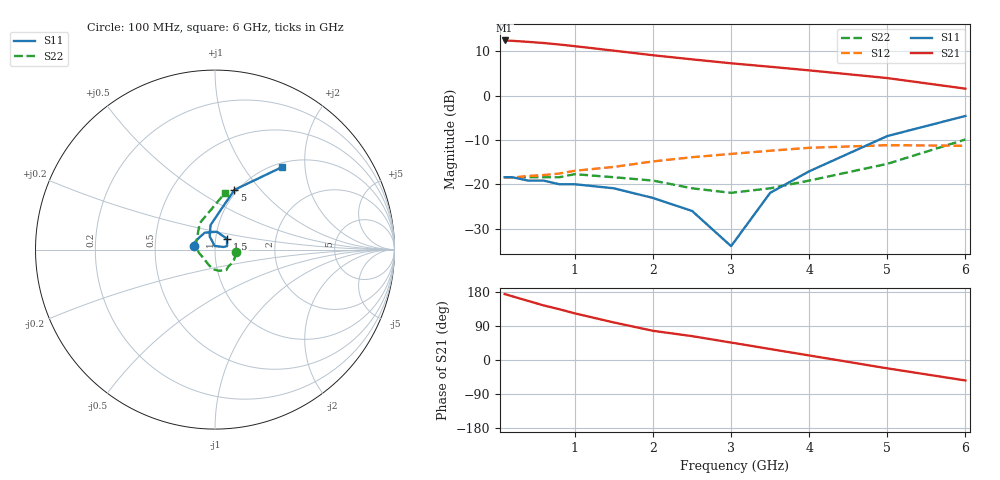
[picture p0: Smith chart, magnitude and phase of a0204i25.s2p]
!  MSA-0204 S AND NOISE PARAMETERS
!  Id=25mA  LAST UPDATED 07-22-92
# ghz s ma r 50
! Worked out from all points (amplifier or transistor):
!   14 points, 100 MHz to 6 GHz, reference 50 ohm
!   highest |S21| = 12.5 dB at 100 MHz (marker M1)
!   |S21| within 3 dB of that: start of sweep to 1.836 GHz
!   unconditionally stable (mu >= 1): start of sweep to end of sweep
!   at 400 MHz: K = 1.21, MAG = 12.4 dB, |S12| = -18.1 dB
!   at 2 GHz: K = 1.22, MAG = 9.2 dB, |S12| = -14.8 dB
!   at 6 GHz: K = 1.21, MAG = 3.7 dB, |S12| = -11.3 dB
!   lowest NFmin = 6.00 dB at 100 MHz
!   S11 on the Smith chart (normalised r, x): 100 MHz: 0.79, +0.03; 1.5 GHz: 1.13, +0.14; 5 GHz: 0.97, +0.73; 6 GHz: 1.08, +1.51
0.1  0.12 170.0  4.2 174.0  0.119 2.0  0.12 -7.0
0.2  0.12 160.0  4.16 168.0  0.119 4.0  0.12 -14.0
0.4  0.11 140.0  4.05 156.0  0.124 6.0  0.12 -29.0
0.6  0.11 121.0  3.93 144.0  0.127 8.0  0.12 -42.0
0.8  0.1 104.0  3.78 134.0  0.132 12.0  0.12 -52.0
1  0.1 84.0  3.62 123.0  0.142 14.0  0.13 -61.0
1.5  0.09 42.0  3.22 99.0  0.157 16.0  0.12 -79.0
2  0.07 16.0  2.86 77.0  0.181 15.0  0.11 -96.0
2.5  0.05 17.0  2.57 63.0  0.202 16.0  0.09 -115.0
3  0.02 95.0  2.32 46.0  0.22 13.0  0.08 -141.0
3.5  0.08 112.0  2.12 29.0  0.239 7.0  0.09 -167.0
4  0.14 100.0  1.93 12.0  0.258 0.0  0.11 171.0
5  0.35 72.0  1.58 -22.0  0.276 -15.0  0.17 120.0
6  0.59 51.0  1.2 -54.0  0.272 -33.0  0.32 80.0
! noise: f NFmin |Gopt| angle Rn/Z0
0.1  6  0.09  1  1.18
0.5  6.3  0.09  5  1.18
1  6.5  0.08  4  1.17
2  6.9  0.06  -2  1.13
